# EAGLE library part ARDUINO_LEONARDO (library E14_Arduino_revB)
Device for representing an Arduino Leonardo board with a footprint in an EAGLE design. Created by Dave Young for Element14. More EAGLE documentation at: http://www.element14.com/community/community/knode/cadsoft_eagle
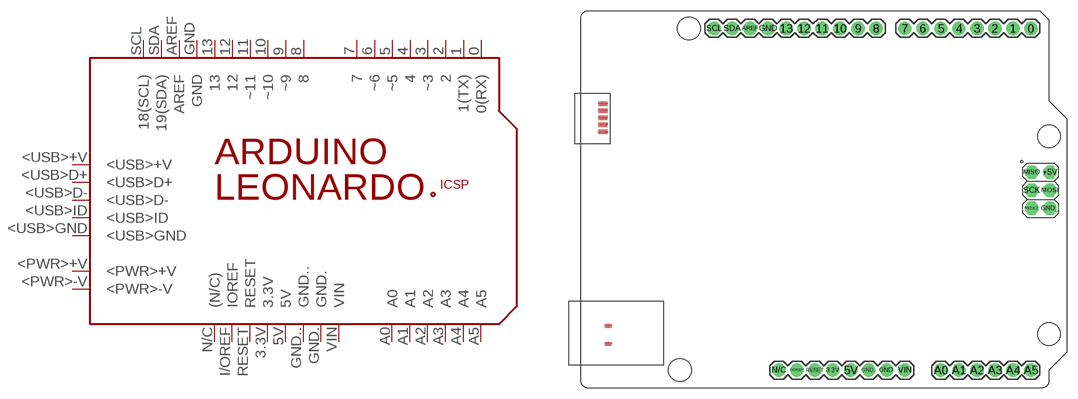
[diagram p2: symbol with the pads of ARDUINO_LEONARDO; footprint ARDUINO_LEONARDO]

Designator prefix PCB

## ARDUINO_LEONARDO  [ARDUINO_LEONARDO]
0  0(RX)
1  1(TX)
2  2
3  ~3
3.3V  3.3V
4  4
5  ~5
5V  5V
6  ~6
7  7
8  8
9  ~9
10  ~10
11  ~11
12  12
13  13
+5V  +5V
<PWR>+V  <PWR>+V
<PWR>-V  <PWR>-V
<USB>+V  <USB>+V
<USB>D+  <USB>D+
<USB>D-  <USB>D-
<USB>GND  <USB>GND
<USB>ID  <USB>ID
A0  A0
A1  A1
A2  A2
A3  A3
A4  A4
A5  A5
AREF  AREF
GND  GND
GND.  GND.
GND..  GND..
GND_  GND_
I/OREF  IOREF
MISO  MISO
MOSI  MOSI
N/C  (N/C)
RESET  RESET
RESET.  RESET.
SCK  SCK
SCL  18(SCL)
SDA  19(SDA)
VIN  VIN

## Footprint ARDUINO_LEONARDO (pad centres in mm)
Footprint for representing an Arduino Leonardo board in an EAGLE schematic. Created by Dave Young for Element14. More EAGLE documentation at: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
drill 1.016 pad 1.88: 0 63.5,50.8; 1 60.96,50.8; 2 58.42,50.8; 3 55.88,50.8; 3.3V 35.56,2.54; 4 53.34,50.8; 5 50.8,50.8; 5V 38.1,2.54; 6 48.26,50.8; 7 45.72,50.8; 8 41.656,50.8; 9 39.116,50.8; 10 36.576,50.8; 11 34.036,50.8; 12 31.496,50.8; 13 28.956,50.8; A0 50.8,2.54; A1 53.34,2.54; A2 55.88,2.54; A3 58.42,2.54; A4 60.96,2.54; A5 63.5,2.54; AREF 23.876,50.8; GND 26.416,50.8; GND. 43.18,2.54; GND.. 40.64,2.54; I/OREF 30.48,2.54; N/C 27.94,2.54; RESET 33.02,2.54; SCL 18.796,50.8; SDA 21.336,50.8; VIN 45.72,2.54
drill 1.016 pad 1.88 octagon: +5V 66.167,30.48; GND_ 66.167,25.4; MISO 63.627,30.48; MOSI 66.167,27.94; RESET. 63.627,25.4; SCK 63.627,27.94
smd 1.016 x 0.508: <PWR>+V 3.861,8.814; <PWR>-V 3.861,6.274
smd 1.27 x 0.635: <USB>+V 3.099,40.157; <USB>D+ 3.099,39.167; <USB>D- 3.099,38.151; <USB>GND 3.099,36.17; <USB>ID 3.099,37.186
hole 3.2 at 66.04,7.62
hole 3.2 at 66.04,35.56
hole 3.2 at 15.24,50.8
hole 3.2 at 13.97,2.54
